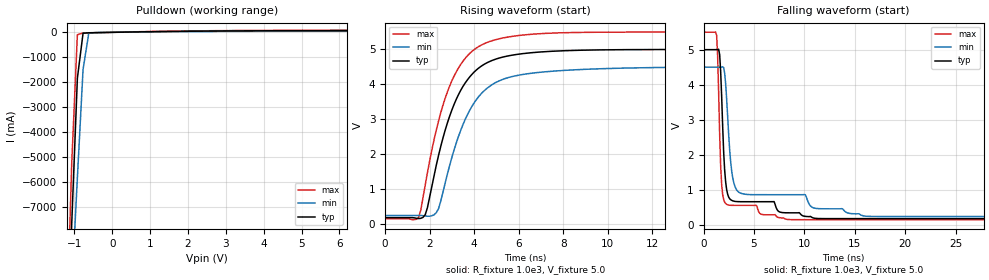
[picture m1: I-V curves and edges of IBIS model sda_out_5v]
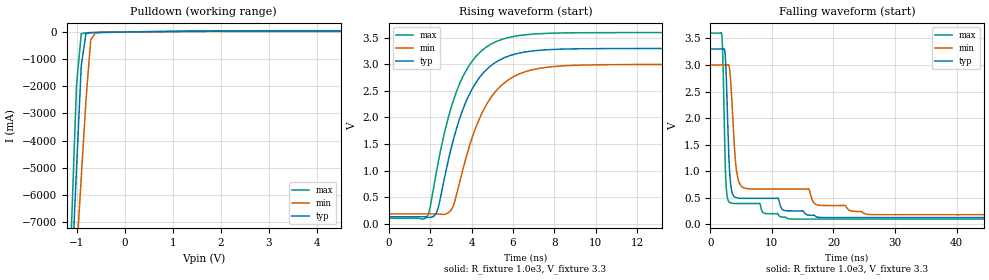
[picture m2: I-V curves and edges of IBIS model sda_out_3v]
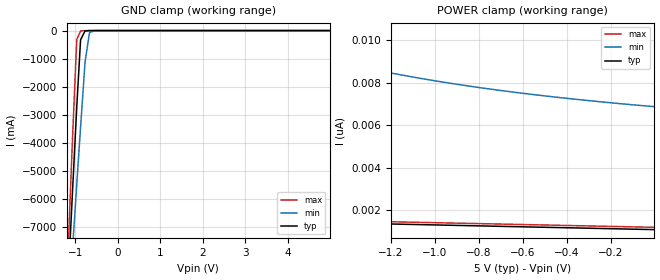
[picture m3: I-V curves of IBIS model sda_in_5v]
|Texas Instruments Incorporated
| 12-Bit, 8-Channel, ADC System Monitor With Temperature Sensor,
| Internal -External ,and I2C Interface
| Marketing part#   Digital Voltage Range   Package-type   #pins
| ADC128D818   3.3V - 5V   TSSOP   16
[IBIS Ver]   4.1
[File name]   adc128d818.ibs
[File Rev]   1.0
[Date]   3/04/2016
[Source]
| Texas Instruments Incorporated.
| Analog-eLab Design Center, HPA
| 12500 TI Blvd
| Dallas, TX -75243
[Notes]   Revision History:
| Rev 1.0: 3/04/2016
| - Initial version of the model
| - Model matched to SPICE simulation
| - C_comp although listed in numerical order of value are
|   obtained from varying PVT conditions. For PVT conditions for
|   each specific value refer the buffer description under
|   respective [Model]. IBIS model user is responsible for using
|   appropriate C_comp to simulate for Signal Integrity.
| - Models was taken from existing LM96080 part.
[Disclaimer]
| This model is designed as an aid for customers of Texas Instruments.
| TI and its licensors and suppliers make no warranties, either expressed
| or implied, with respect to this  model, including the warranties of
| merchantability or fitness for a particular purpose. The model is
| provided solely on an "as is" basis. The entire risk as to its quality
| and performance is with the customer.
[Copyright]
(C) Copyright 2016 Texas Instruments Incorporated.All rights reserved
|   ADC128D818PW
[Component]   ADC128D818PW
[Manufacturer]   TI
[Package]   |16 TSSOP - PW package
|   typ   min   max
R_pkg   0.10   0.03   0.12
L_pkg   3nH   1.8nH   4.2nH
C_pkg   0.45pF   0.36pF   0.55pF
[Pin]   signal_name   model_name   R_pin   L_pin   C_pin
1   VREF   NC   0.12257  4.21681n  0.54750p
2   SDA   SDA   0.08395  2.54847n  0.38017p
3   SCL   SCL   0.06407  2.13675n  0.35667p
4   GND   GND   0.03723  1.96911n  0.38462p
5   V+   POWER   0.03693  1.87723n  0.39469p
6   _INT   INT   0.06382  2.13186n  0.35810p
7   A0   A0   0.09439  2.76575n  0.39489p
8   A1   A1   0.12166  4.19768n  0.55073p
9   IN7   NC   0.11641  4.09373n  0.55089p
10   IN6   NC   0.09105  2.70374n  0.40046p
11   IN5   NC   0.07605  2.38914n  0.37893p
12   IN4   NC   0.06630  2.18947n  0.36575p
13   IN3   NC   0.06388  2.14055n  0.36239p
14   IN2   NC   0.06853  2.23566n  0.36820p
15   IN1   NC   0.08052  2.48561n  0.38435p
16   IN0   NC   0.10419  3.83702n  0.53452p
[Model Selector] SDA
sda_in_3v   3.3V  digital Input
sda_in_5v   5.5V  digital Input
sda_out_3v   3.3V  digital Open_sink
sda_out_5v   5.5V  digital Open_sink
[Model Selector] SCL
scl_3v   3.3V  digital Input
scl_5v   5.5V  digital Input
[Model Selector] INT
int_out_3v   3.3V  digital Output
int_out_5v   5.5V  digital Output
[Model Selector] A0
a0_3v   3.3V  digital Input
a0_5v   5.5V  digital Input
[Model Selector] A1
a1_3v   3.3V  digital Input
a1_5v   5.5V  digital Input
| Models and submodels in the file (12): sda_out_5v (Open_sink), sda_out_3v (Open_sink), sda_in_5v (Input), sda_in_3v (Input), scl_5v (Input), scl_3v (Input), a1_5v (Input), a1_3v (Input), a0_5v (Input), a0_3v (Input), int_out_5v (Output), int_out_3v (Output)
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[Model] sda_out_5v
Model_type Open_sink
Vmeas = 0.4V
Cref = 0.0pF
Rref = 1.0e3
Vref = 5.0V
C_comp   1.61pF   0.89pF   1.90pF
[Voltage Range]   5.0V   4.5V   5.5V
[Temperature Range]   25.0   125.0   -40.0
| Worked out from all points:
|   slope of the pulldown table from 0 to 0.75 V, typ, clamps not added: 38.1 ohm
|   rising waveform, R_fixture 1.0e3, V_fixture 5.0: 20-80 % time 1.48ns typ, 1.54ns min, 1.43ns max; typ from 0.17 V to 5 V
|   falling waveform, R_fixture 1.0e3, V_fixture 5.0: 20-80 % time 484ps typ, 846ps min, 350ps max; typ from 5 V to 0.17 V
[Pulldown]
-5V       -161.4A    -126.1A    -200.9A
-1.22V    -13.68A    -14.84A    -12.86A
-1.07V    -7.679A    -10.29A    -5.265A
-920mV    -1.833A    -5.819A    -93.47mA
-770mV    -35.61mA   -1.481A    -29.03mA
-620mV    -17.46mA   -40.2mA    -22.66mA
-305mV    -8.646mA   -5.711mA   -11.55mA
2.875V    53.3mA     36.61mA    67.8mA
10V       68.75mA    48.56mA    87.6mA
[Rising Waveform]
R_fixture=1.0e3
V_fixture=5.0
V_fixture_min=4.5
V_fixture_max=5.5
0s        170.3mV    231.6mV    140.1mV
1.5ns     143.1mV    231.6mV    175.3mV
1.8ns     251.7mV    222.3mV    1.104V
2.4ns     1.955V     427.6mV    2.945V
3ns       3.26V      1.898V     4.1V
3.6ns     4.037V     2.99V      4.743V
4.7ns     4.653V     3.941V     5.227V
6.5ns     4.9V       4.31V      5.43V
15.5ns    4.998V     4.493V     5.498V
99.95ns   5V         4.5V       5.5V
[Falling Waveform]
R_fixture=1.0e3
V_fixture=5.0
V_fixture_min=4.5
V_fixture_max=5.5
0s        5V         4.5V       5.5V
1.3ns     5V         4.5V       5.411V
1.4ns     5.001V     4.5V       4.816V
1.7ns     4.379V     4.5V       1.679V
2.1ns     1.541V     4.321V     637.4mV
2.7ns     710.2mV    1.773V     551mV
3.2ns     659.9mV    1.035V     548.5mV
8.2ns     337.1mV    854mV      152.3mV
16.5ns    170.3mV    233.9mV    140.1mV
99.95ns   170.3mV    231.6mV    140.1mV
[Ramp]
R_load = 1.0e3
dV/dt_r   2.897826E0/1.4E-9   2.561001E0/1.6E-9   3.215929E0/1.4E-9
dV/dt_f   2.897831E0/5E-10   2.561007E0/9E-10   3.215933E0/3E-10
[Model] sda_out_3v
Model_type Open_sink
Vmeas = 0.4V
Cref = 0.0pF
Rref = 1.0e3
Vref = 3.3V
C_comp   1.61pF   0.89pF   1.90pF
[Voltage Range]   3.3V   3.0V   3.6V
[Temperature Range]   25.0   125.0   -40.0
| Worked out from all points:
|   slope of the pulldown table from 0 to 0.495 V, typ, clamps not added: 43.7 ohm
|   rising waveform, R_fixture 1.0e3, V_fixture 3.3: 20-80 % time 1.59ns typ, 1.65ns min, 1.54ns max; typ from 0.129 V to 3.3 V
|   falling waveform, R_fixture 1.0e3, V_fixture 3.3: 20-80 % time 672ps typ, 1.41ns min, 453ps max; typ from 3.3 V to 0.129 V
[Pulldown]
-3.3V     -95.44A    -76.45A    -116.9A
-1.201V   -12.92A    -14.27A    -11.9A
-1.102V   -8.955A    -11.27A    -6.876A
-1.003V   -5.047A    -8.285A    -1.953A
-904.2mV  -1.227A    -5.354A    -63.83mA
-805.2mV  -59.07mA   -2.486A    -29.17mA
-706.2mV  -20.09mA   -279.5mA   -23.46mA
-607.2mV  -15.02mA   -30.77mA   -20.14mA
1.996V    31.68mA    20.03mA    44.45mA
6.6V      35.4mA     22.46mA    49.81mA
[Rising Waveform]
R_fixture=1.0e3
V_fixture=3.3
V_fixture_min=3.0
V_fixture_max=3.6
0s        129.5mV    183.6mV    101.8mV
1.9ns     119.6mV    183.6mV    159.5mV
2.4ns     308.6mV    180.9mV    1.173V
3ns       1.395V     247.6mV    2.165V
3.8ns     2.357V     1.333V     2.924V
4.7ns     2.892V     2.228V     3.321V
5.6ns     3.128V     2.656V     3.485V
6.8ns     3.245V     2.884V     3.564V
12ns      3.298V     2.996V     3.598V
99.95ns   3.3V       3V         3.6V
[Falling Waveform]
R_fixture=1.0e3
V_fixture=3.3
V_fixture_min=3.0
V_fixture_max=3.6
0s        3.3V       3V         3.6V
1.9ns     3.3V       3V         3.538V
2.5ns     3.038V     3V         892.4mV
2.9ns     1.648V     3.009V     452.8mV
3.4ns     677.1mV    2.54V      401.7mV
4ns       514.5mV    1.312V     394.6mV
4.6ns     495mV      817.2mV    394.2mV
8.8ns     491mV      665.7mV    209.4mV
26ns      129.5mV    185.6mV    101.8mV
99.95ns   129.5mV    183.6mV    101.8mV
[Ramp]
R_load = 1.0e3
dV/dt_r   1.902307E0/1.6E-9   1.689856E0/1.6E-9   2.098945E0/1.5E-9
dV/dt_f   1.90231E0/6E-10   1.68986E0/1.4E-9   2.098947E0/5E-10
[Model] sda_in_5v
Model_type Input
Vinh = 3.5V
Vinl = 1.5V
C_comp   1.61pF   0.89pF   1.90pF
[Voltage Range]   5.0V   4.5V   5.5V
[Temperature Range]   25.0   125.0   -40.0
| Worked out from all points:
|   GND clamp passes 1 mA (typ) near -0.64 V on its own axis
[GND Clamp]
-5V       -123.9A    -96.98A    -153.9A
-1.175V   -9.121A    -10.37A    -8.099A
-1.07V    -5.878A    -7.904A    -4.016A
-965mV    -2.716A    -5.471A    -323.5mA
-875mV    -328.9mA   -3.437A    -14.52mA
-770mV    -14.3mA    -1.128A    -1.547mA
-665mV    -1.225mA   -74.04mA   -105.9uA
-560mV    -78.44uA   -7.068mA   -3.614uA
4.99V     1.095nA    0A         1.093nA
[POWER Clamp]
-5V       2.251nA    48.01nA    2.3nA
-1.97V    1.533nA    10.54nA    1.636nA
-1.91V    1.52nA     10.33nA    1.623nA
-1.82V    1.5nA      10.03nA    1.603nA
-1.67V    1.466nA    9.571nA    1.57nA
-1.46V    1.419nA    9.017nA    1.524nA
-1.265V   1.376nA    8.578nA    1.482nA
-1.055V   1.33nA     8.175nA    1.436nA
-800mV    1.273nA    7.765nA    1.38nA
-560mV    1.22nA     7.443nA    1.327nA
-305mV    1.164nA    7.155nA    1.271nA
-5mV      1.098nA    6.868nA    1.206nA
